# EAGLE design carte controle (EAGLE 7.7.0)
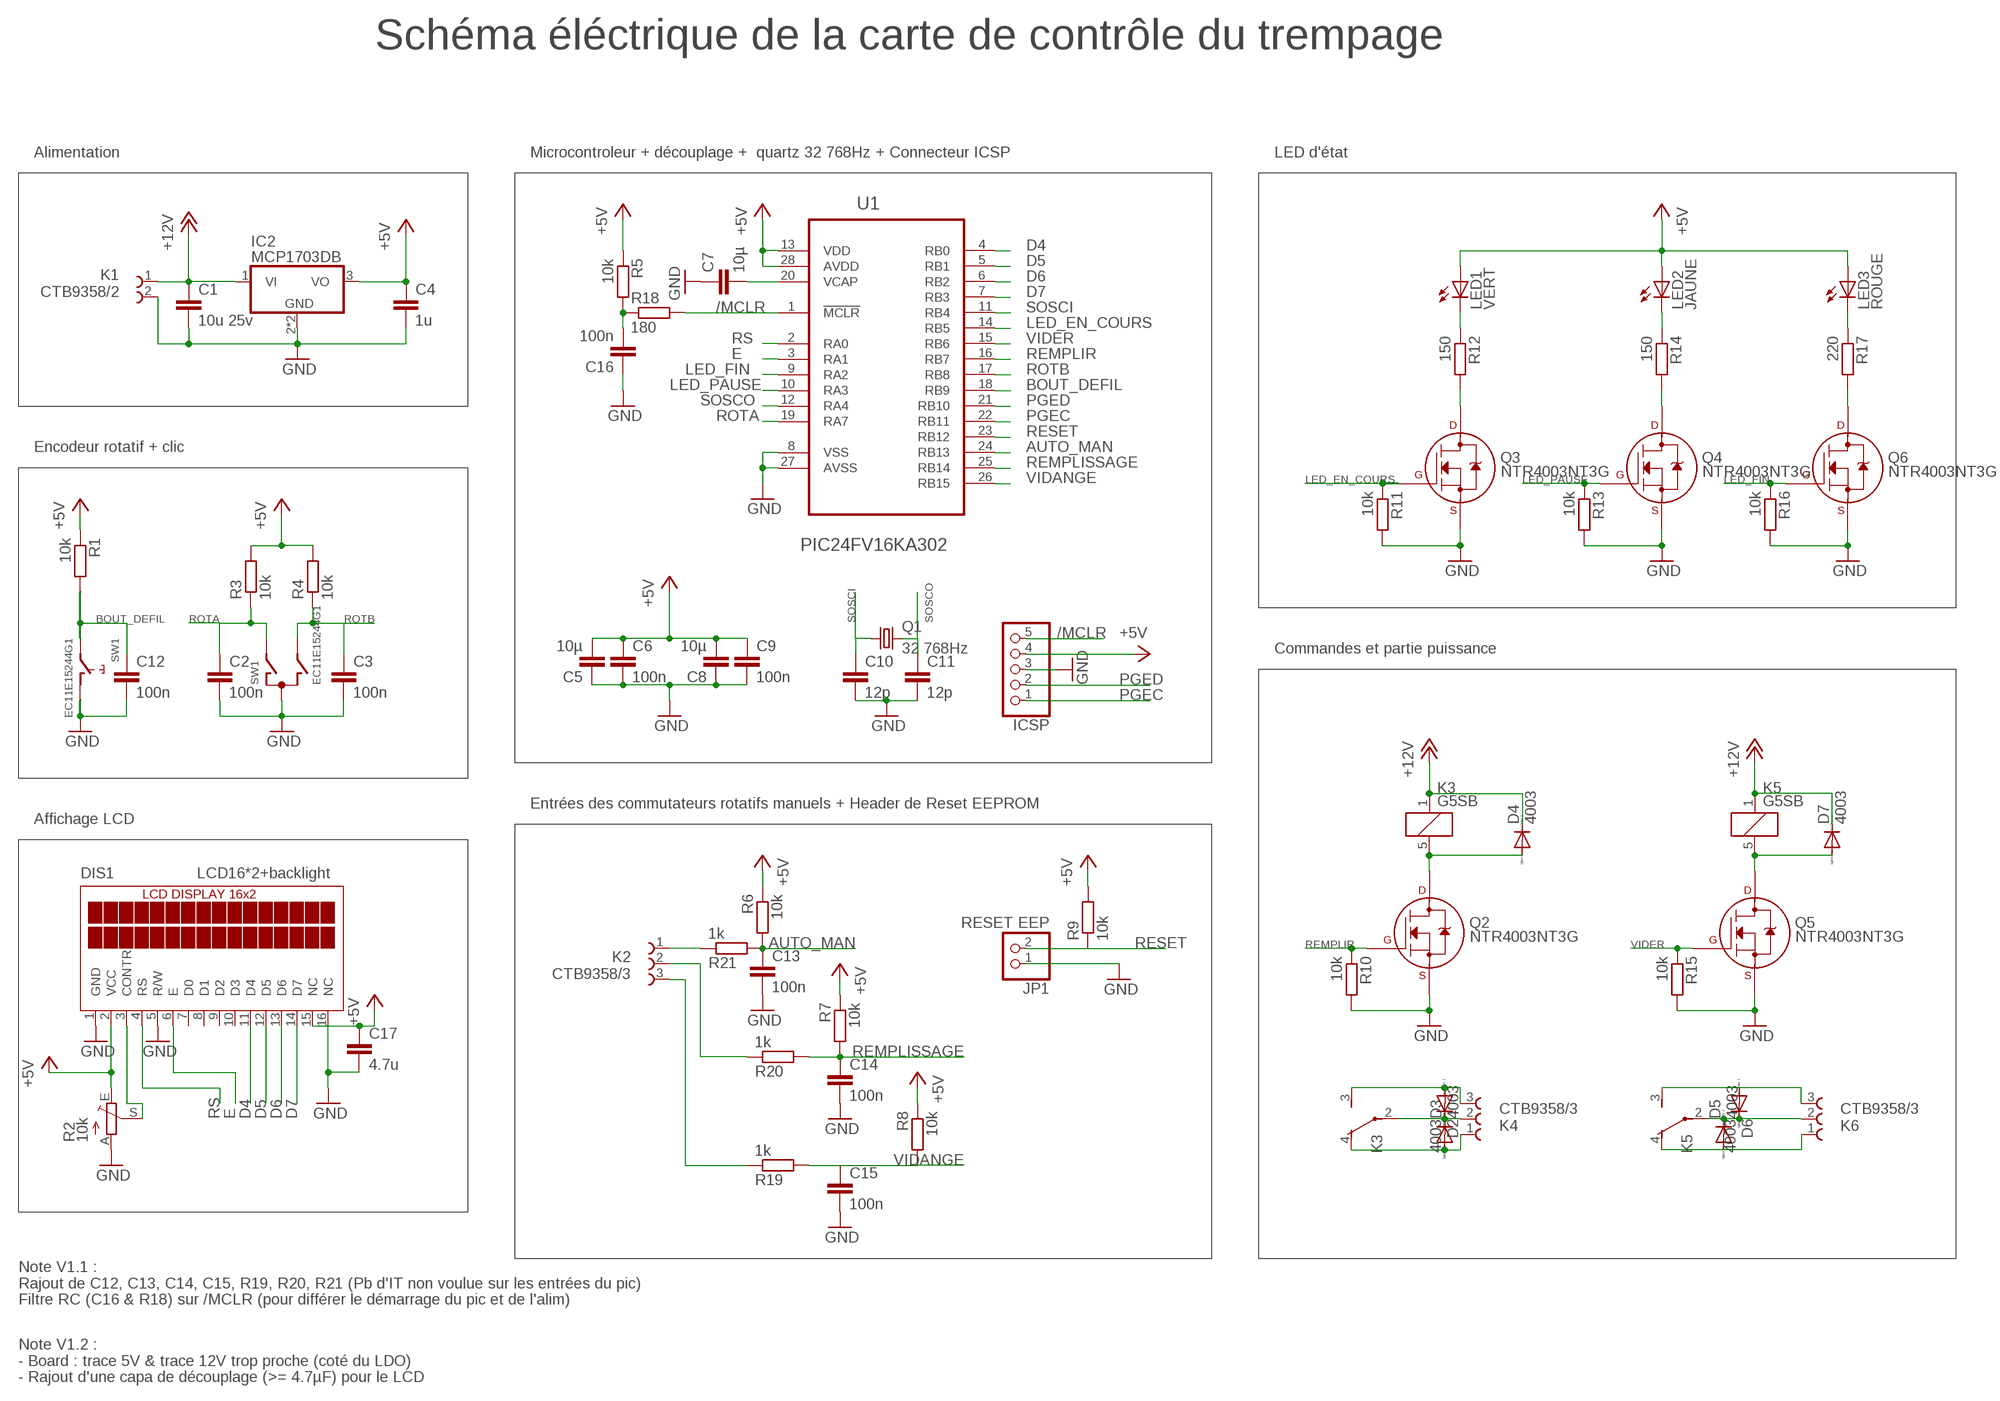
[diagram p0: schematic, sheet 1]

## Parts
C1  10u 25v  C-EUC1210  [C1210]
C2  100n  C-EUC0805  [C0805]
C3  100n  C-EUC0805  [C0805]
C4  1u  C-EUC0805  [C0805]
C5  10µ  C-EUC1206  [C1206]
C6  100n  C-EUC0805  [C0805]
C7  10µ  C-EUC1206  [C1206]
C8  10µ  C-EUC1206  [C1206]
C9  100n  C-EUC0805  [C0805]
C10  12p  C-EUC0805  [C0805]
C11  12p  C-EUC0805  [C0805]
C12  100n  C-EUC0805  [C0805]
C13  100n  C-EUC0805  [C0805]
C14  100n  C-EUC0805  [C0805]
C15  100n  C-EUC0805  [C0805]
C16  100n  C-EUC0805  [C0805]
C17  4.7u  C-EUC1206  [C1206]
D2  4003  DIODE-MELF-MLL41  [MELF-MLL41]
D3  4003  DIODE-MELF-MLL41  [MELF-MLL41]
D4  4003  DIODE-MELF-MLL41  [MELF-MLL41]
D5  4003  DIODE-MELF-MLL41  [MELF-MLL41]
D6  4003  DIODE-MELF-MLL41  [MELF-MLL41]
D7  4003  DIODE-MELF-MLL41  [MELF-MLL41]
DIS1  LCD16*2+backlight  TUXGR_16X2_R2  [TUXGR_16X2_R2]
IC2  MCP1703DB  [SOT223]
ICSP  PINHD-1X5  [1X05]
JP1  RESET EEP  PINHD-1X2  [1X02]
K1  CTB9358/2  691313510002  [691313510002]
K2  CTB9358/3  691313510003  [691313510003]
K3  G5SB  [G5SB]
K4  CTB9358/3  691313510003  [691313510003]
K5  G5SB  [G5SB]
K6  CTB9358/3  691313510003  [691313510003]
LED1  VERT  LED5MM  [LED5MM]
LED2  JAUNE  LED5MM  [LED5MM]
LED3  ROUGE  LED5MM  [LED5MM]
Q1  32 768Hz  CRYSTALTC26V  [TC26V]
Q2  NTR4003NT3G  2N7000_SOT23  [SOT-23]
Q3  NTR4003NT3G  2N7000_SOT23  [SOT-23]
Q4  NTR4003NT3G  2N7000_SOT23  [SOT-23]
Q5  NTR4003NT3G  2N7000_SOT23  [SOT-23]
Q6  NTR4003NT3G  2N7000_SOT23  [SOT-23]
R1  10k  R-EU_M0805  [M0805]
R2  10k  TRIM_EU-S64W  [S64W]
R3  10k  R-EU_M0805  [M0805]
R4  10k  R-EU_M0805  [M0805]
R5  10k  R-EU_M0805  [M0805]
R6  10k  R-EU_M0805  [M0805]
R7  10k  R-EU_M0805  [M0805]
R8  10k  R-EU_M0805  [M0805]
R9  10k  R-EU_M0805  [M0805]
R10  10k  R-EU_M0805  [M0805]
R11  10k  R-EU_M0805  [M0805]
R12  150  R-EU_M0805  [M0805]
R13  10k  R-EU_M0805  [M0805]
R14  150  R-EU_M0805  [M0805]
R15  10k  R-EU_M0805  [M0805]
R16  10k  R-EU_M0805  [M0805]
R17  220  R-EU_M0805  [M0805]
R18  180  R-EU_M0805  [M0805]
R19  1k  R-EU_M0805  [M0805]
R20  1k  R-EU_M0805  [M0805]
R21  1k  R-EU_M0805  [M0805]
SW1  EC11E15244G1  EC12E_SW  [ALPS_EC12E_SW]
U1  PIC24FV16KA302  PIC24FV32KA302-I/SO  [SOIC127P1030X265-28N]

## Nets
+5V: C4.1 C5.2 C6.1 C8.2 C9.1 C17.1 DIS1.2(VCC) DIS1.15(NC) IC2.3(VO) ICSP.4 LED1.A LED2.A LED3.A R1.1 R2.E R3.2 R4.2 R5.1 R6.1 R7.1 R8.1 R9.2 U1.13(VDD) U1.28(AVDD)
+12V: C1.1 D4.C D7.C IC2.1(VI) K1.1 K3.1 K5.1
/MCLR: ICSP.5 R18.2 U1.1(!MCLR)
AUTO_MAN: C13.1 R6.2 R21.2 U1.24(RB13)
BOUT_DEFIL: C12.1 R1.2 SW1.E U1.18(RB9)
D4: DIS1.11(D4) U1.4(RB0)
D5: DIS1.12(D5) U1.5(RB1)
D6: DIS1.13(D6) U1.6(RB2)
D7: DIS1.14(D7) U1.7(RB3)
E: DIS1.6(E) U1.3(RA1)
GND: C1.2 C2.2 C3.2 C4.2 C5.1 C6.2 C7.1 C8.1 C9.2 C10.2 C11.2 C12.2 C13.2 C14.2 C15.2 C16.1 C17.2 DIS1.1(GND) DIS1.5(R/W) DIS1.16(NC) IC2.2(GND) IC2.4(GND) ICSP.3 JP1.1 K1.2 Q2.2(S) Q3.2(S) Q4.2(S) Q5.2(S) Q6.2(S) R2.A R10.2 R11.2 R13.2 R15.2 R16.2 SW1.C SW1.D U1.8(VSS) U1.27(AVSS)
LED_EN_COURS: Q3.1(G) R11.1 U1.14(RB5)
LED_FIN: Q6.1(G) R16.1 U1.9(RA2)
LED_PAUSE: Q4.1(G) R13.1 U1.10(RA3)
N$1: Q6.3(D) R17.2
N$2: D5.C D6.C K5.2(U:P) K6.2
N$3: C7.2 U1.20(VCAP)
N$4: D7.A K5.5 Q5.3(D)
N$5: LED1.K(C) R12.1
N$6: C16.2 R5.2 R18.1
N$7: K2.3 R19.1
N$8: K2.2 R20.1
N$9: LED2.K(C) R14.1
N$10: Q4.3(D) R14.2
N$11: Q3.3(D) R12.2
N$12: LED3.K(C) R17.1
N$13: D6.A K5.3(U:S) K6.3
N$14: D4.A K3.5 Q2.3(D)
N$15: D5.A K5.4(U:O) K6.1
N$16: D2.A K3.3(U:S) K4.3
N$17: D2.C D3.C K3.2(U:P) K4.2
N$18: D3.A K3.4(U:O) K4.1
N$19: K2.1 R21.1
N$24: DIS1.3(CONTR) R2.S
PGEC: ICSP.1 U1.22(RB11)
PGED: ICSP.2 U1.21(RB10)
REMPLIR: Q2.1(G) R10.1 U1.16(RB7)
REMPLISSAGE: C14.1 R7.2 R20.2 U1.25(RB14)
RESET: JP1.2 R9.1 U1.23(RB12)
ROTA: C2.1 R3.1 SW1.A U1.19(RA7)
ROTB: C3.1 R4.1 SW1.B U1.17(RB8)
RS: DIS1.4(RS) U1.2(RA0)
SOSCI: C10.1 Q1.1 U1.11(RB4)
SOSCO: C11.1 Q1.2 U1.12(RA4)
VIDANGE: C15.1 R8.2 R19.2 U1.26(RB15)
VIDER: Q5.1(G) R15.1 U1.15(RB6)
Unconnected: DIS1.7(D0) DIS1.8(D1) DIS1.9(D2) DIS1.10(D3) SW1.GND1(G) SW1.GND2(G)

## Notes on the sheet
- Schéma éléctrique de la carte de contrôle du trempage
- Alimentation | Microcontroleur + découplage +  quartz 32 768Hz + Connecteur ICSP | LED d'état
- Encodeur rotatif + clic
- Commandes et partie puissance
- Entrées des commutateurs rotatifs manuels + Header de Reset EEPROM
- Affichage LCD
- Note V1.1 :
  Rajout de C12, C13, C14, C15, R19, R20, R21 (Pb d'IT non voulue sur les entrées du pic)
  Filtre RC (C16 & R18) sur /MCLR (pour différer le démarrage du pic et de l'alim)
- Note V1.2 :
  - Board : trace 5V & trace 12V trop proche (coté du LDO)
  - Rajout d'une capa de découplage (>= 4.7µF) pour le LCD

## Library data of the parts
C1-C9 C12-C17 = resistor:C-EU: CAPACITOR, European symbol
C10 C11 = rcl:C-EU: CAPACITOR, European symbol
D2-D7 = diode:DIODE-: DIODE
DIS1 = display-lcd:TUXGR_16X2_R2: Tuxgraphics LCD display 16x2 characters reflective, without background light Source: tuxgr_12x2_r2.pdf; OC_FARNELL: unknown; OC_NEWARK: unknown
IC2 = linear:MCP1703: 250 mA, 16V, Low Quiescent Current LDO Regulator Source: http://ww1.microchip.com/downloads/en/DeviceDoc/22049b.pdf
ICSP = pinhead:PINHD-1X5: PIN HEADER
JP1 = pinhead:PINHD-1X2: PIN HEADER
K1 = Terminal_Blocks_Connectors_rev15e:691313510002: WR-TBL Serie 313 - 5.08 mm Close Horizontal PCB Header , 2 Pins=>Code : Con_TBL_Pluggable_5.08_PCB_THT_Simple_H_691313510002
K2 K4 K6 = Terminal_Blocks_Connectors_rev15e:691313510003: WR-TBL Serie 313 - 5.08 mm Close Horizontal PCB Header , 3 Pins=>Code : Con_TBL_Pluggable_5.08_PCB_THT_Simple_H_691313510003 Details see: http://katalog.we-online.de/en/em/691_313_510_0xx Created 2014-06-25, Karrer Zheng 2014 (C) Würth Elektronik
K3 K5 = relay:G5SB: Compact Single-pole Relay for Switching 5 A Source: http://www.omron.com/ecb/products/pry/121/g5sb.html; OC_FARNELL: unknown; OC_NEWARK: unknown
LED1-LED3 = led:LED: LED
Q1 = crystal:CRYSTAL: CRYSTAL; OC_FARNELL: unknown; OC_NEWARK: unknown
Q2-Q6 = transistors:2N700*: 2N7000, 2N7002, NDS7002A N-channel enhancement mode MOSFET
R1 R3-R21 = resistor:R-EU_: RESISTOR, European symbol
R2 = pot:TRIM_EU-: POTENTIOMETER
SW1 = switch-alps:EC12E_SW: ALPS rotary Encoder EC12E series with switch; MPN: EC12E2424407; OC_FARNELL: 1520813; OC_NEWARK: 74M1068
U1 = PIC24:PIC24FV32KA302-I/SO: 16-bit Microcontrollers a,SOIC-28; MPN: PIC24FV32KA302-I/SO; OC_FARNELL: 1898815; OC_NEWARK: 13T4818; PACKAGE: SOIC-28; SUPPLIER: MICROCHIP

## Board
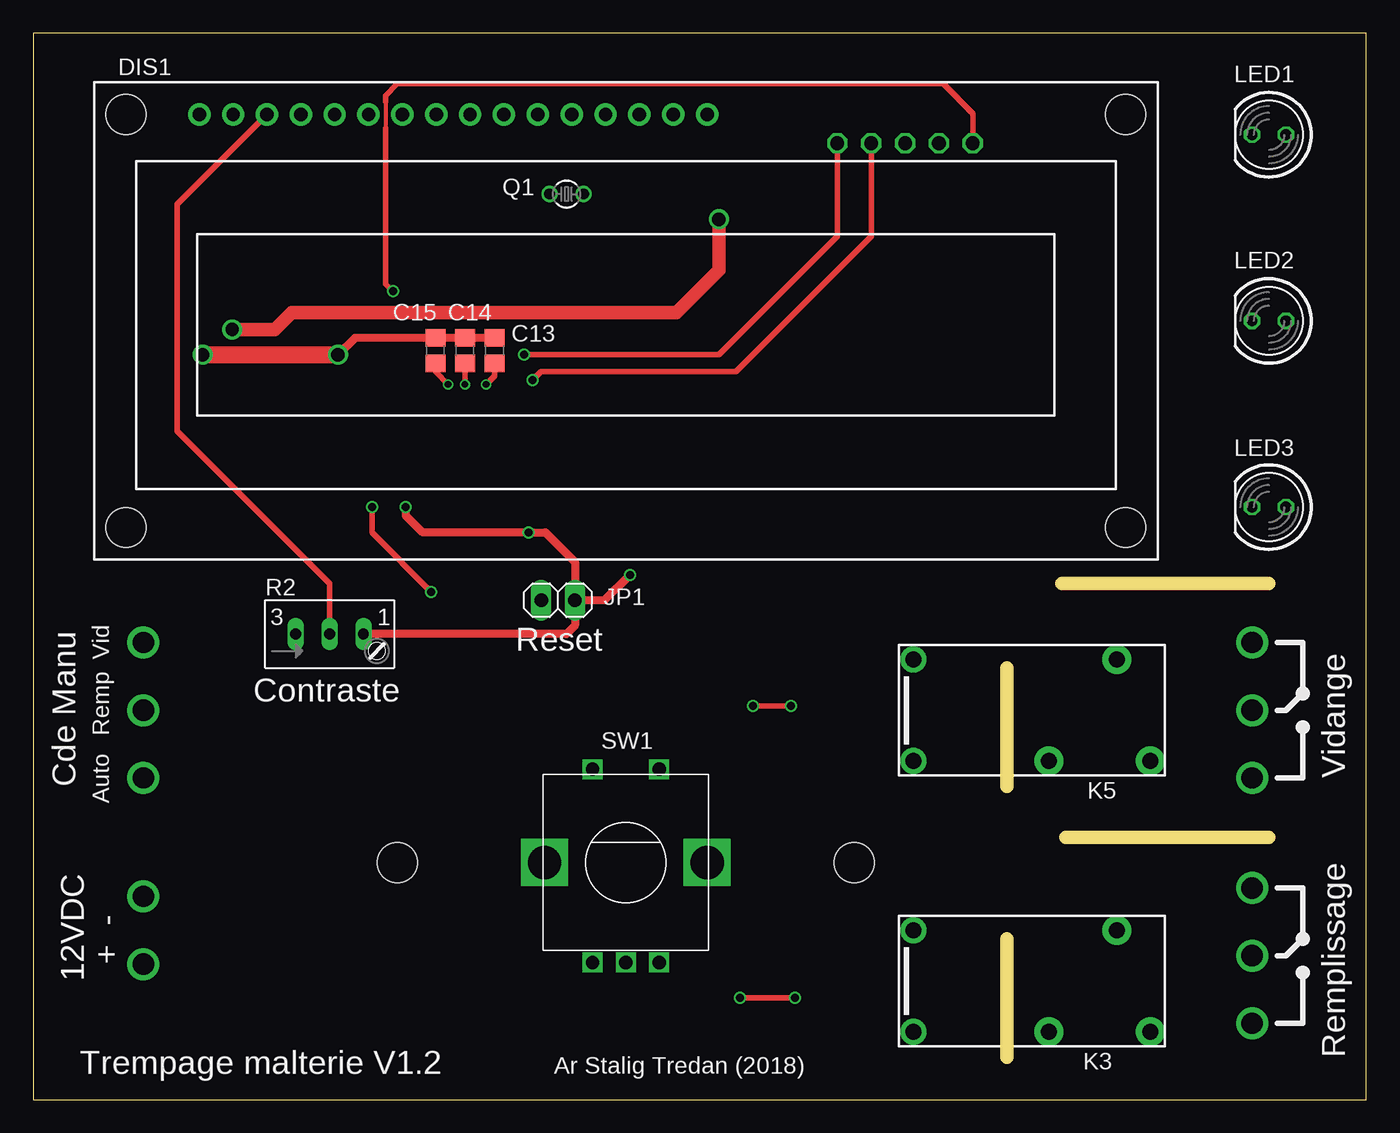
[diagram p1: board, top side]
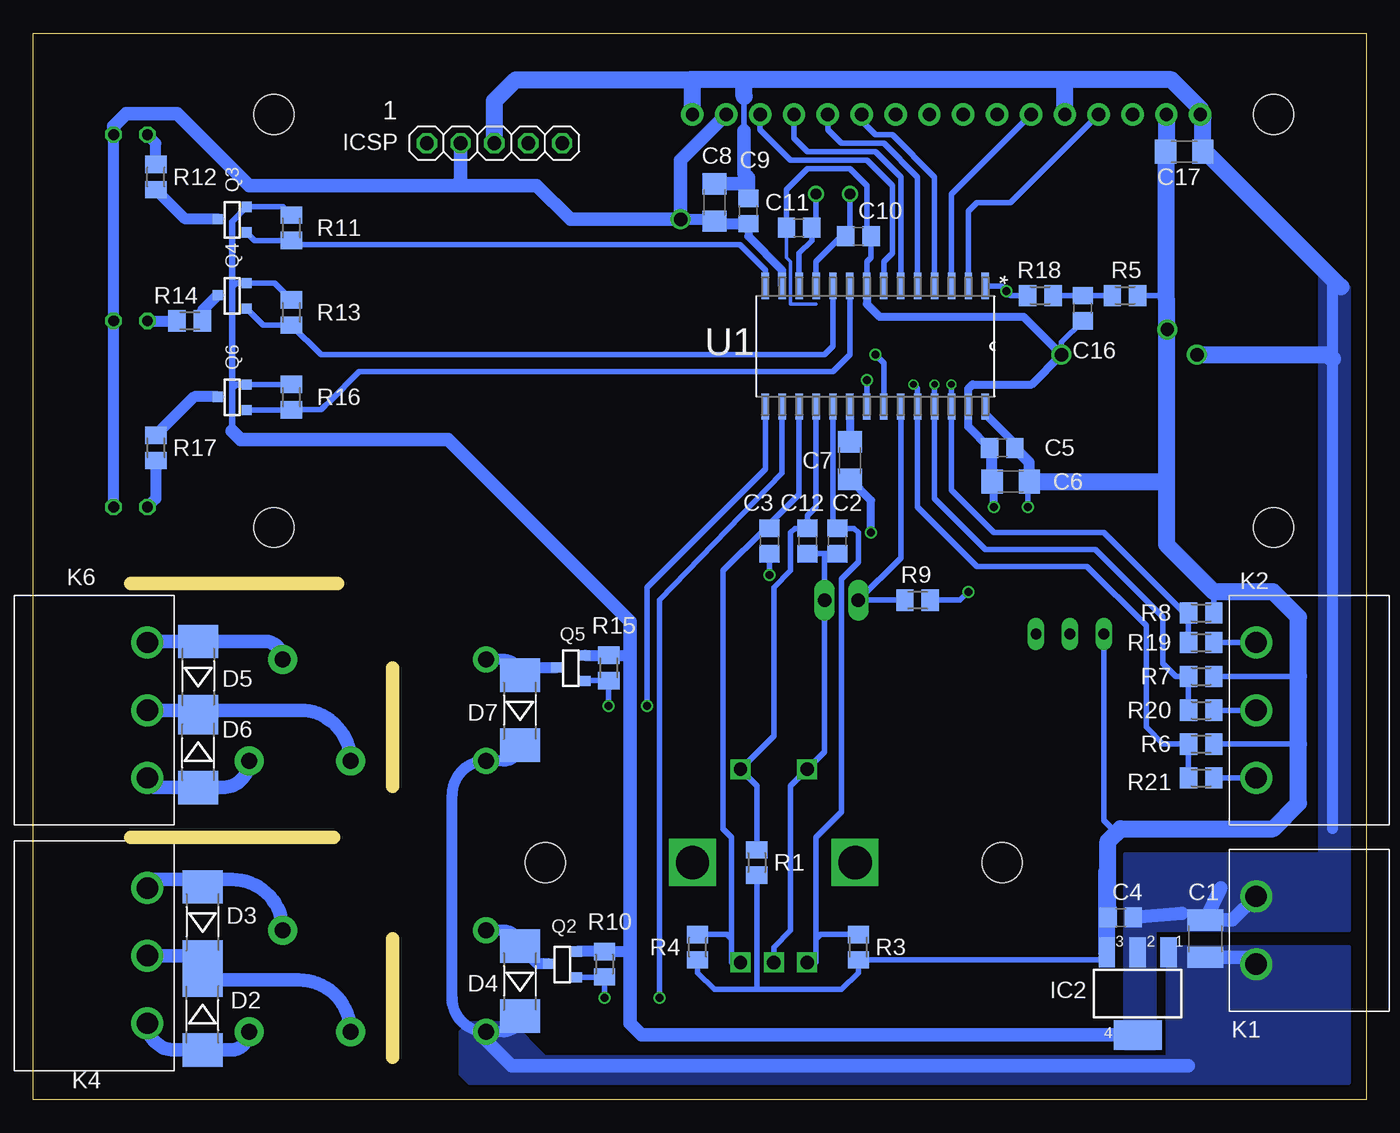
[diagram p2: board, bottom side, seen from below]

Size 100 x 80 mm. Coordinates in mm from the lower left corner, seen from the top.
Outline: 0,0 100,0 100,80 0,80 0,0
Copper layers (1*16): Top 0.035559375mm / dielectric 1.6mm / Bottom 0.035559375mm
Design rules "jlcpcb2layer": minimum track width 5mil, minimum drill 12mil, track to track 5mil, track to pad 5mil, pad to pad 5mil, via to via 5mil, smd to smd 5mil, copper to edge 8mil, drill to drill 6mil, minimum pad ring 5mil, minimum via ring 3mil, stop-mask expansion 2.5mil, vias tented up to drill 0mil, thermal gap 10mil
Holes 3 mm at 61.59,17.78 27.3,17.78
Milling: 4 lines

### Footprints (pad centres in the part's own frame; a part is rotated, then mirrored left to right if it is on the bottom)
C1210 = smd 1.6 x 2.7: 1 -1.4,0; 2 1.4,0
C0805 = smd 1.3 x 1.5: 1 -0.95,0; 2 0.95,0
C1206 = smd 1.6 x 1.8: 1 -1.4,0; 2 1.4,0
MELF-MLL41 = smd 2.5 x 3: A 2.625,0; C -2.625,0
TUXGR_16X2_R2 = drill 1 pad 1.676: 1 -32,15.5; 2 -29.46,15.5; 3 -26.92,15.5; 4 -24.38,15.5; 5 -21.84,15.5; 6 -19.3,15.5; 7 -16.76,15.5; 8 -14.22,15.5; 9 -11.68,15.5; 10 -9.14,15.5; 11 -6.6,15.5; 12 -4.06,15.5; 13 -1.52,15.5; 14 1.02,15.5; 15 3.56,15.5; 16 6.1,15.5 | hole 3: -37.5,-15.5; 37.5,-15.5; -37.5,15.5; 37.5,15.5
SOT223 = smd 1.219 x 2.235: 1 -2.311,-3.099; 2 0,-3.099; 3 2.311,-3.099 | smd 3.6 x 2.2: 4 0,3.099
1X05 = drill 1.016 octagon: 1 -5.08,0; 2 -2.54,0; 3 0,0; 4 2.54,0; 5 5.08,0
1X02 = drill 1.016 long: 1 -1.27,0; 2 1.27,0
691313510002 = drill 1.6: 1 -5.08,0; 2 0,0
691313510003 = drill 1.6: 1 -5.08,0; 2 0,0; 3 5.08,0
G5SB = drill 1.2 pad 1.93: 1 7.62,3.81; 5 7.62,-3.81 | drill 1.2 pad 2.184: 2 -2.54,3.81; 3 -10.16,3.81; 4 -7.62,-3.81
LED5MM = drill 0.813 octagon: A -1.27,0; K 1.27,0
TC26V = drill 0.813: 1 -1.27,0; 2 1.27,0
SOT-23 = smd 0.762 x 0.762: 1 -0.979,-1.101; 2 0.94,-1.101; 3 0.025,1.067
M0805 = smd 1.3 x 1.6: 1 -0.95,0; 2 0.95,0
S64W = drill 0.813 long: A 2.54,1.27; E -2.54,1.27; S 0,1.27
ALPS_EC12E_SW = drill 1 square: A -2.5,-7.5; B 2.5,-7.5; C 0,-7.5; D -2.5,7; E 2.5,7 | drill 2.5 square: GND1 -6.1,0; GND2 6.1,0
SOIC127P1030X265-28N = smd 1.981 x 0.559: 1 -4.521,8.255; 2 -4.521,6.985; 3 -4.521,5.715; 4 -4.521,4.445; 5 -4.521,3.175; 6 -4.521,1.905; 7 -4.521,0.635; 8 -4.521,-0.635; 9 -4.521,-1.905; 10 -4.521,-3.175; 11 -4.521,-4.445; 12 -4.521,-5.715; 13 -4.521,-6.985; 14 -4.521,-8.255; 15 4.521,-8.255; 16 4.521,-6.985; 17 4.521,-5.715; 18 4.521,-4.445; 19 4.521,-3.175; 20 4.521,-1.905; 21 4.521,-0.635; 22 4.521,0.635; 23 4.521,1.905; 24 4.521,3.175; 25 4.521,4.445; 26 4.521,5.715; 27 4.521,6.985; 28 4.521,8.255

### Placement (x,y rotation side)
C1  12.06,12.06 90 bottom
C2  39.69,41.91 270 bottom
C3  44.77,41.91 270 bottom
C4  18.41,13.65 0 bottom
C5  26.67,46.35 0 bottom
C6  27.3,48.9 180 bottom
C7  38.73,47.94 90 bottom
C8  48.9,67.31 270 bottom
C9  46.35,66.67 90 bottom
C10  38.1,64.77 0 bottom
C11  42.55,65.41 180 bottom
C12  41.91,41.91 270 bottom
C13  34.61,56.2 90 top
C14  32.38,56.2 90 top
C15  30.16,56.2 90 top
C16  21.27,59.37 90 bottom
C17  13.65,71.12 0 bottom
D2  87.31,6.35 270 bottom
D3  87.31,13.34 90 bottom
D4  63.5,8.89 90 bottom
D5  87.63,31.75 90 bottom
D6  87.63,26.04 270 bottom
D7  63.5,29.21 90 bottom
DIS1  44.45,58.42 0 top
IC2  17.14,7.94 180 bottom
ICSP  65.41,71.75 180 bottom
JP1  39.37,37.47 180 top
K1  8.26,15.24 90 bottom
K2  8.26,29.21 90 bottom
K3  73.66,8.89 180 top
K4  91.44,10.79 270 bottom
K5  73.66,29.21 180 top
K6  91.44,29.21 270 bottom
LED1  92.71,72.39 180 top
LED2  92.71,58.42 180 top
LED3  92.71,44.45 180 top
Q1  40.01,67.94 0 top
Q2  60.33,10.16 90 bottom
Q3  85.09,66.04 90 bottom
Q4  85.09,60.33 90 bottom
Q5  59.69,32.38 90 bottom
Q6  85.09,52.7 90 bottom
R1  45.72,17.78 90 bottom
R2  22.23,33.66 0 top
R3  38.1,11.43 270 bottom
R4  50.16,11.43 270 bottom
R5  18.1,60.33 180 bottom
R6  12.38,26.67 180 bottom
R7  12.38,31.75 180 bottom
R8  12.38,36.51 180 bottom
R9  33.66,37.47 0 bottom
R10  57.15,10.16 90 bottom
R11  80.64,65.41 90 bottom
R12  90.81,69.22 270 bottom
R13  80.64,59.05 90 bottom
R14  88.27,58.42 0 bottom
R15  56.83,32.38 90 bottom
R16  80.64,52.7 90 bottom
R17  90.81,48.9 90 bottom
R18  24.45,60.33 180 bottom
R19  12.38,34.29 180 bottom
R20  12.38,29.21 180 bottom
R21  12.38,24.13 180 bottom
SW1  44.45,17.78 0 top
U1  36.83,56.52 270 bottom

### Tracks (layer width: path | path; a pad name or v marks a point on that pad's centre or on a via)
+5V  (via drill 0.6, 1)
  Top 0.406: v29.84,38.1 25.4,42.55 v25.4,44.45
  Top 1.016: v14.92,57.78 18.1,57.78 19.37,59.05 48.26,59.05 51.44,62.23 v51.44,66.04
  Bottom 0.406: v25.4,44.45 25.4,46.23 | 48.71,65.72 C8.2 | R4.2 50.16,9.53 48.9,8.26 45.72,8.26 | 45.72,8.26 39.37,8.26 38.1,9.53 R3.2 20.01,10.48 IC2.3 | R7.1 5.08,31.75 | R6.1 5.08,26.67 | R1.1 45.72,8.26 | R2.E 19.68,20.95 18.73,20 | R9.2 30.48,37.47 v29.84,38.1 | R5.1 15.31,60.33 14.99,60.01 | R8.1 11.43,38.1
  Bottom 0.61: 25.4,46.23 C5.2 | C6.1 26.36,49.22 28.57,51.44 U1.28 | U1.13 43.81,62.23 46.35,64.77 C9.1
  Bottom 0.813: LED3.A LED2.A LED1.A | C6.1 25.27,47.81 C5.2 | 48.71,65.72 C9.1 | v51.44,66.04 49.02,66.04 C8.2
  Bottom 1.016: v14.92,57.78 14.92,59.3 14.99,59.37 | DIS1.15 51.44,70.5 v51.44,66.04 59.69,66.04 62.23,68.58 68.26,68.58 | LED1.A 93.98,73.03 93.03,73.98 89.22,73.98 83.82,68.58 68.26,68.58 | ICSP.4 67.94,68.9 68.26,68.58
  Bottom 1.27: 14.99,46.67 14.99,59.37 14.99,60.01 14.99,71.06 C17.1 14.99,71.18 DIS1.2 | 14.99,46.67 14.99,41.66 11.43,38.1 6.99,38.1 5.08,36.2 5.08,31.75 5.08,26.67 5.08,22.23 6.99,20.32 18.41,20.32 18.73,20 19.36,19.37 C4.1 19.46,17.05 IC2.3 | C5.2 15.31,46.35 14.99,46.67
+12V
  Bottom 0.813: D4.C arc90 64.69,5.08 K3.1 arc90 68.58,7.62 68.58,22.86 arc90 K5.1 64.69,25.4 arc-90 D7.C
  Bottom 1.016: 13.34,2.54 64.14,2.54 66.04,4.45 K3.1 | C1.1 8.76,10.66 K1.1
  pour Bottom (no thermals): 1.27,11.43 14.92,11.43 14.92,3.17 61.59,3.17 64.14,5.71 67.31,5.71 67.94,5.08 67.94,1.91 67.31,1.27 1.27,1.27
/MCLR  (via drill 0.6)
  Top 0.305: 26.43,74.85 26.43,72.87
  Top 0.406: 26.43,74.85 26.43,75.33 27.3,76.2 68.26,76.2 70.48,73.98 ICSP.5 | 26.43,72.87 26.43,61.2 v26.99,60.64
  Bottom 0.406: U1.1 27.38,61.04 v26.99,60.64 26.67,60.33 R18.2
AUTO_MAN  (via drill 0.5)
  Top 0.406: C13.1 34.61,54.29 v33.97,53.66
  Bottom 0.406: v33.97,53.66 33.66,53.34 U1.24 33.66,44.45 29.21,40.01 20.95,40.01 16.51,35.56 16.51,27.94 15.24,26.67 R6.2 R21.2
BOUT_DEFIL
  Bottom 0.406: U1.18 41.27,44.45 41.91,43.81 C12.1 42.87,42.86 43.18,42.55 43.18,39.69 44.45,38.42 44.45,27.28 SW1.E | 46.99,24.82 SW1.E | SW1.E 45.72,23.55 R1.2
D4
  Bottom 0.406: U1.4 32.38,69.22 35.56,72.39 36.83,72.39 37.85,73.41 DIS1.11
D5
  Bottom 0.406: U1.5 33.66,69.22 36.2,71.75 39.37,71.75 40.39,72.78 DIS1.12
D6
  Bottom 0.406: U1.6 34.92,69.22 36.83,71.12 41.91,71.12 42.93,72.14 DIS1.13
D7
  Bottom 0.406: U1.7 36.2,62.87 35.56,63.5 35.56,68.58 37.47,70.48 43.18,70.48 45.47,72.78 DIS1.14
E
  Bottom 0.406: DIS1.6 31.11,67.94 U1.3
GND  (via drill 0.6, 1)
  Top 0.61: JP1.1 40.64,35.56 40.01,34.92 R2.A | v27.94,44.45 27.94,43.81 29.21,42.55 v37.15,42.55 38.42,42.55 40.64,40.33 JP1.1 | C13.2 C14.2 C15.2 24.13,57.15 v22.86,55.88 | JP1.1 42.86,37.47 v44.77,39.37
  Top 1.27: v12.7,55.88 v22.86,55.88
  Bottom 0.254: C11.2 43.49,63.18 43.18,62.87 43.18,59.69 41.27,59.69
  Bottom 0.406: R13.2 81.91,61.27 Q4.2 | Q6.2 80.66,53.65 R16.2 | Q3.2 81.27,66.98 R11.2 | C11.2 43.49,68.27 41.91,69.85 38.73,69.85 37.47,68.58 37.47,64.45 C10.2 37.15,63.19 37.15,63.18 37.47,62.87 U1.8 | 13.84,13.97 C1.2 | SW1.C 44.45,11.43 43.18,12.7 43.18,23.55 SW1.D 40.64,26.09 JP1.1 40.64,40.96 | v22.86,55.88 22.86,56.84 C16.1 | 41.59,40.96 C12.2 40.64,40.96 | C2.2 40.64,40.96 | v44.77,39.37 C3.2 | 46.67,72.71 46.67,75.25
  Bottom 0.5: 85.09,60.96 85.09,65.88 Q3.2 | 85.09,60.96 85.09,53.34 | 85.09,53.34 85.09,50.16 | Q6.2 84.78,53.65 85.09,53.34 | Q4.2 84.78,61.27 85.09,60.96
  Bottom 0.61: C5.1 27.94,46.23 v27.94,44.45 | C6.2 29.84,50.48 U1.27 29.84,53.34 29.53,53.66 25.08,53.66 v22.86,55.88 25.72,58.74 36.51,58.74 37.47,59.69 U1.8 | C7.1 37.15,44.95 v37.15,42.55
  Bottom 0.813: 2.54,20.32 2.54,55.56 2.54,60.96 1.91,60.96 | Q2.2 R10.2 55.24,11.11 | C5.1 28.07,48.71 C6.2 | Q5.2 arc90 58.58,33.34 R15.2 arc90 R15.2 55.24,33.34
  Bottom 1.016: 85.09,50.16 84.45,49.53 68.9,49.53 55.24,35.88 55.24,33.34 55.24,11.11 55.24,5.71 54.37,4.84 IC2.4 | 10.93,15.88 C1.2 10.03,13.46 K1.2 | 13.84,13.97 C4.2 | 46.67,72.71 46.67,69.48 46.35,69.16 46.35,68.26 | C9.2 46.35,68.26 | C8.1 46.8,68.71 46.35,68.26
  Bottom 1.27: v12.7,55.88 2.86,55.88 2.54,55.56 | 22.86,76.52 14.61,76.52 12.45,74.36 DIS1.1 12.25,73.72 C17.2 12.06,71.12 1.91,60.96 | 22.86,76.52 46.67,76.52 | 46.67,76.52 50.8,76.52 | DIS1.16 50.55,76.27 50.8,76.52 | DIS1.5 22.61,76.27 22.86,76.52 | 46.67,75.25 46.67,76.52 | ICSP.3 65.41,74.93 63.82,76.52 50.8,76.52
  pour Bottom (no thermals): 1.27,12.7 15.88,12.7 15.88,3.81 18.1,3.81 18.1,18.41 3.49,18.41 3.49,62.87 1.27,60.96
LED_EN_COURS
  Bottom 0.406: Q3.1 83.38,64.45 R11.1 80.33,64.14 46.99,64.14 45.09,62.23 U1.14
LED_FIN
  Bottom 0.406: Q6.1 80.67,51.73 R16.1 78.42,51.76 78.11,52.07 77.79,52.39 75.56,54.61 40.01,54.61 38.73,55.88 U1.9
LED_PAUSE
  Bottom 0.406: Q4.1 82.75,58.1 R13.1 78.42,55.88 40.64,55.88 40.01,56.52 U1.10
N$1
  Bottom 0.813: Q6.3 87.92,52.73 R17.2
N$2
  Bottom 0.813: D6.C D5.C
  Bottom 1.016: 88.35,29.21 88.27,29.2 | 88.27,29.2 D5.C arc90 88.18,29.21 80.01,29.21 arc90 K5.2 | D6.C 88.27,27.94 | K6.2 arc-90 K6.2 88.27,29.2
N$3
  Bottom 0.61: U1.20 C7.2
N$4
  Bottom 0.813: K5.5 64.69,33.02 arc90 D7.A arc90 62.92,32.41 Q5.3
N$5
  Bottom 0.813: R12.1 90.81,71.75 LED1.K
N$6
  Bottom 0.406: R5.2 C16.2 R18.1
N$7
  Bottom 0.406: K2.3 R19.1
N$8
  Bottom 0.406: K2.2 R20.1
N$9
  Bottom 0.813: LED2.K R14.1
N$10
  Bottom 0.813: R14.2 87.31,59.19 Q4.3
N$11
  Bottom 0.813: Q3.3 88.61,66.06 R12.2
N$12
  Bottom 0.813: R17.1 90.81,45.09 LED3.K
N$13
  Bottom 1.016: K5.3 arc90 85.81,23.41 D6.A 90.72,23.41 arc90 K6.3
N$14
  Bottom 0.813: D4.A arc-90 64.69,12.7 K3.5 | 63.36,11.52 D4.A | Q2.3 62.17,10.19 D4.A
N$15
  Bottom 1.016: K5.4 arc-90 82.64,34.38 D5.A 91.36,34.38 arc90 K6.1
N$16
  Bottom 1.016: K4.3 arc-90 89.45,3.73 D2.A 85.17,3.73 arc-90 K3.3
N$17
  Bottom 1.016: 87.55,9.84 D2.C | D3.C 87.63,10.79 | 87.63,10.79 D2.C | 87.95,9.21 arc-90 87.63,9.53 D2.C | K3.2 arc-90 80.09,8.97 D2.C | 87.63,10.79 K4.2
N$18
  Bottom 0.813: D3.A 88.9,16.51
  Bottom 1.016: K3.4 arc-90 85.09,16.51 88.9,16.51 90.81,16.51 arc-90 K4.1
N$19
  Bottom 0.406: K2.1 R21.1
N$24
  Top 0.406: R2.S 22.23,38.73 10.79,50.16 10.79,67.19 DIS1.3
PGEC  (via drill 0.6)
  Top 0.406: v36.83,55.88 51.44,55.88 60.33,64.77 ICSP.1
  Bottom 0.406: U1.22 36.2,55.24 v36.83,55.88
PGED  (via drill 0.6)
  Top 0.406: v37.47,53.98 38.1,54.61 52.7,54.61 62.87,64.77 ICSP.2
  Bottom 0.406: U1.21 v37.47,53.98
REMPLIR  (via drill 0.6)
  Top 0.406: v53.02,7.62 v57.15,7.62
  Bottom 0.406: U1.16 43.81,46.99 53.02,37.47 v53.02,7.62 | Q2.1 57.18,9.18 R10.1 v57.15,7.62
REMPLISSAGE  (via drill 0.5)
  Top 0.406: v32.38,53.66 C14.1
  Bottom 0.406: v32.38,53.66 U1.25 32.38,45.09 28.57,41.27 20.32,41.27 15.24,36.2 15.24,32.7 14.29,31.75 R7.2 R20.2
RESET
  Bottom 0.406: R9.1 JP1.2 34.92,40.64 U1.23
ROTA
  Bottom 0.406: U1.19 40.01,43.18 C2.1 38.42,42.86 38.1,42.55 38.1,40.32 39.37,39.05 39.37,21.59 41.27,19.68 41.27,12.06 | SW1.A 41.27,10.28 41.27,12.06 | R3.1 40.96,12.38 41.27,12.06
ROTB
  Bottom 0.406: U1.17 42.55,45.4 44.77,43.18 C3.1 45.09,42.86 48.26,39.69 48.26,20.32 47.62,19.68 47.62,12.06 | SW1.B 47.62,10.28 47.62,12.06 | R4.1 47.94,12.38 47.62,12.06
RS
  Bottom 0.406: U1.2 29.84,66.67 29.21,67.31 26.68,67.31 DIS1.4
SOSCI
  Bottom 0.406: Q1.1 38.73,65.08 C10.1 39.37,64.77 41.27,62.87 U1.11
SOSCO
  Bottom 0.406: Q1.2 41.27,65.72 C11.1 41.59,64.45 42.55,63.5 U1.12
VIDANGE  (via drill 0.5)
  Top 0.406: C15.1 30.16,54.61 v31.11,53.66
  Bottom 0.406: v31.11,53.66 U1.26 31.11,45.72 27.94,42.55 19.68,42.55 13.65,36.51 R8.2 R19.2
VIDER  (via drill 0.6)
  Top 0.406: v56.83,29.53 v53.98,29.53
  Bottom 0.406: U1.15 45.09,47.31 53.98,38.42 v53.98,29.53 | Q5.1 arc90 58.56,31.43 R15.1 v56.83,29.53

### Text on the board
tNames: Reset | Vid | Contraste | Remp | Vidange | Cde Manu | Auto | + - | 12VDC | Remplissage | Trempage malterie V1.2 | Ar Stalig Tredan (2018)
bNames: 1

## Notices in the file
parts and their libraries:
Terminal_Blocks_Connectors_rev15e: Copyright: Würth Elektronik
